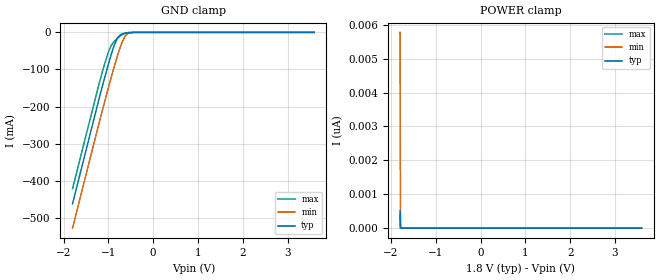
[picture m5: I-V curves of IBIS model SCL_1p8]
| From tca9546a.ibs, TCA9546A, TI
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|   Model
[Model]   SCL_1p8
Model_type   Input
Vinl = 0.54
Vinh = 1.26
|   typ   min   max
C_comp   3.557pF   3.453pF   3.722pF
[Voltage Range]   1.8   1.65   1.95
[Temperature Range]   27   125   -40
[Power Clamp Reference]   1.8   1.65   1.95
[GND Clamp Reference]   -0   -0   -0
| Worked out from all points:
|   GND clamp passes 1 mA (typ) near -0.59 V on its own axis
[GND Clamp]
|   Voltage   I(typ)   I(min)   I(max)
-1.8V     -462.2mA   -527.5mA   -421.4mA
-1.238V   -193.3mA   -259mA     -153mA
-1.087V   -124mA     -188.9mA   -86.26mA
-995.4mV  -83.9mA    -147.4mA   -51.61mA
-941.4mV  -61.65mA   -123.5mA   -36.73mA
-876.6mV  -37.47mA   -95.56mA   -25.44mA
-795.6mV  -15.15mA   -62.53mA   -15.69mA
-698.4mV  -4.427mA   -28.15mA   -6.92mA
-628.2mV  -1.752mA   -10.68mA   -2.858mA
-558mV    -565.9uA   -2.553mA   -840.4uA
-363.6mV  -7.899uA   -26.51uA   -6.982uA
3.595V    0A         0A         0A
[POWER Clamp]
|   Voltage   I(typ)   I(min)   I(max)
-1.8V     511.7pA    5.778nA    356.1pA
-1.789V   0A         0A         0A
-1.784V   0A         0A         0A
3.595V    0A         0A         0A
